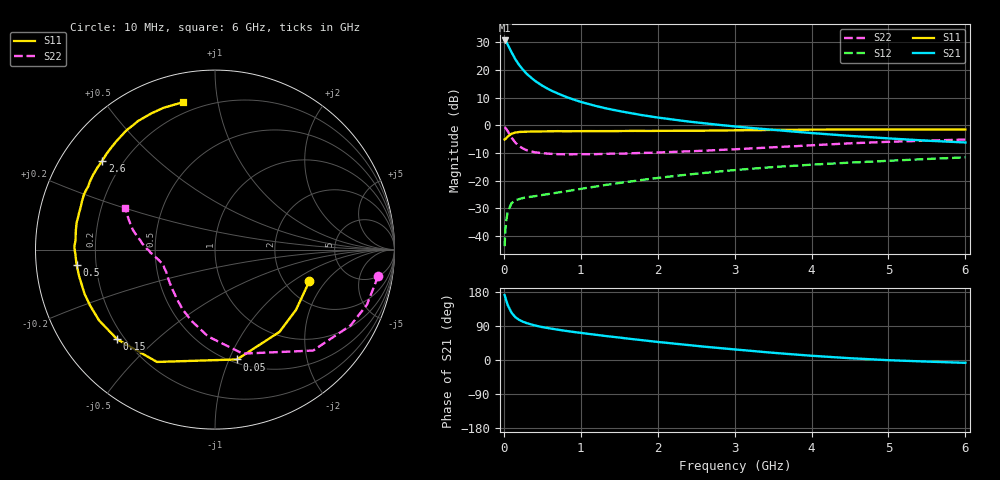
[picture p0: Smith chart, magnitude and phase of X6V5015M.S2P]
! SIEMENS Small Signal Semiconductors
! BFP193W
! Si NPN RF Bipolar Junction Transistor in SOT343
! VCE = 0.5 V  IC = 15 mA
! Common Emitter S-Parameters:  April 1994
# GHz  S  MA  R  50
!  f  S11  S21  S12  S22
! GHz  MAG  ANG  MAG  ANG  MAG  ANG  MAG  ANG
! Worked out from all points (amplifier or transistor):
!   40 points, 10 MHz to 6 GHz, reference 50 ohm
!   highest |S21| = 30.7 dB at 10 MHz (marker M1)
!   |S21| within 3 dB of that: start of sweep to 77.45 MHz
!   unconditionally stable (mu >= 1): 850.3 MHz to end of sweep
!   at 200 MHz: K = 0.33, MSG = 24.2 dB, |S12| = -26.7 dB
!   at 1.5 GHz: K = 1.22, MAG = 10.2 dB, |S12| = -20.9 dB
!   at 6 GHz: K = 1.09, MAG = 0.8 dB, |S12| = -11.6 dB
!   S11 on the Smith chart (normalised r, x): 10 MHz: 2.71, -1.37; 50 MHz: 0.53, -1.07; 150 MHz: 0.17, -0.38; 500 MHz: 0.13, -0.05; 2.6 GHz: 0.12, +0.34; 6 GHz: 0.14, +0.80
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0.01  0.5546 -18.4  34.3 171.4  0.0065 83.0  0.9208 -9.2
0.02  0.5626 -36.7  33.53 164.6  0.0129 75.1  0.9004 -20.0
0.03  0.5825 -51.9  32.42 157.6  0.0183 69.4  0.8656 -29.2
0.05  0.6241 -78.7  28.95 145.0  0.0269 58.3  0.7845 -45.8
0.1  0.7044 -117.3  21.01 124.8  0.0391 41.9  0.5998 -75.1
0.15  0.7395 -137.5  15.66 112.9  0.0438 33.7  0.4852 -94.6
0.2  0.7569 -148.6  12.29 105.8  0.0463 30.9  0.4185 -108.1
0.25  0.7626 -155.9  10.09 100.8  0.0484 29.2  0.38 -118.1
0.3  0.7674 -161.2  8.466 97.2  0.0497 28.7  0.3527 -125.8
0.4  0.7712 -168.6  6.452 91.3  0.0521 29.4  0.3255 -136.5
0.5  0.7759 -173.8  5.209 86.9  0.0548 31.5  0.313 -143.7
0.6  0.778 -177.8  4.357 83.3  0.0577 33.4  0.3052 -149.1
0.8  0.7786 176.0  3.302 77.0  0.0636 37.1  0.2988 -155.7
1.1  0.7853 168.8  2.432 69.0  0.0746 41.4  0.3002 -161.6
1.3  0.7846 164.7  2.068 63.9  0.0824 43.4  0.3034 -163.9
1.6  0.7897 159.1  1.708 56.8  0.0944 45.2  0.3091 -166.8
2.2  0.7964 148.6  1.27 43.6  0.1201 45.6  0.3302 -172.1
2.6  0.7997 141.8  1.09 35.3  0.1371 44.7  0.3467 -175.6
3.2  0.8163 132.4  0.9 24.4  0.1629 41.8  0.3807 179.2
4.5  0.8377 115.0  0.643 4.7  0.2112 33.6  0.4721 166.3
5.5  0.8387 106.3  0.527 -4.2  0.2454 27.8  0.5282 158.2
6  0.8402 102.1  0.489 -7.5  0.2631 25.0  0.5527 155.0
